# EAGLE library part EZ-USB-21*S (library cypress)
Microcontroller with USB port
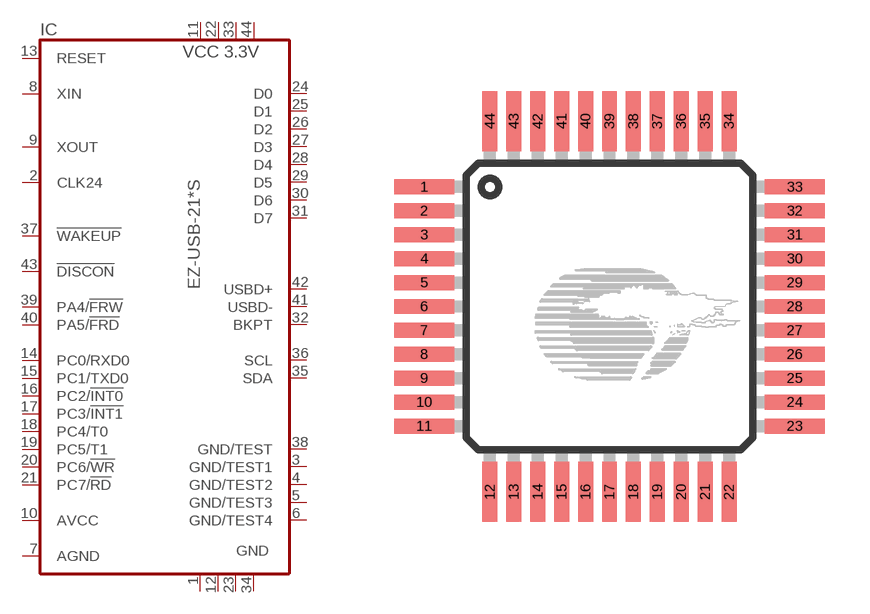
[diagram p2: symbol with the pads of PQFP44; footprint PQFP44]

Designator prefix IC

## EZ-USB-2125S (OC_FARNELL: unknown; OC_NEWARK: unknown), EZ-USB-2126S (OC_FARNELL: unknown; OC_NEWARK: unknown), EZ-USB-2135S (OC_FARNELL: unknown; OC_NEWARK: unknown), EZ-USB-2136S (OC_FARNELL: unknown; OC_NEWARK: unknown)  [PQFP44]
1  GND  pwr
2  CLK24  out
3  GND/TEST1  pwr
4  GND/TEST2  pwr
5  GND/TEST3  pwr
6  GND/TEST4  pwr
7  AGND  pwr
8  XIN  in
9  XOUT  out
10  AVCC  pwr
11  VCC3.3  pwr
12  GND  pwr
13  RESET  in
14  PC0/RXD0
15  PC1/TXD0
16  PC2/!INT0
17  PC3/!INT1
18  PC4/T0
19  PC5/T1
20  PC6/!WR
21  PC7/!RD
22  VCC3.3  pwr
23  GND  pwr
24  D0  hiz
25  D1  hiz
26  D2  hiz
27  D3  hiz
28  D4  hiz
29  D5  hiz
30  D6  hiz
31  D7  hiz
32  BKPT  out
33  VCC3.3  pwr
34  GND  pwr
35  SDA  oc
36  SCL  oc
37  !WAKEUP  in
38  GND/TEST  pwr
39  PA4/!FRW
40  PA5/!FRD
41  USBD-  hiz
42  USBD+  hiz
43  !DISCON  out
44  VCC3.3  pwr

## Footprint PQFP44 (pad centres in mm)
Plastic Quad Flat Package
smd 2 x 0.5: 1 -6.2,4; 2 -6.2,3.2; 3 -6.2,2.4; 4 -6.2,1.6; 5 -6.2,0.8; 6 -6.2,0; 7 -6.2,-0.8; 8 -6.2,-1.6; 9 -6.2,-2.4; 10 -6.2,-3.2; 11 -6.2,-4; 23 6.2,-4; 24 6.2,-3.2; 25 6.2,-2.4; 26 6.2,-1.6; 27 6.2,-0.8; 28 6.2,0; 29 6.2,0.8; 30 6.2,1.6; 31 6.2,2.4; 32 6.2,3.2; 33 6.2,4
smd 0.5 x 2: 12 -4,-6.2; 13 -3.2,-6.2; 14 -2.4,-6.2; 15 -1.6,-6.2; 16 -0.8,-6.2; 17 0,-6.2; 18 0.8,-6.2; 19 1.6,-6.2; 20 2.4,-6.2; 21 3.2,-6.2; 22 4,-6.2; 34 4,6.2; 35 3.2,6.2; 36 2.4,6.2; 37 1.6,6.2; 38 0.8,6.2; 39 0,6.2; 40 -0.8,6.2; 41 -1.6,6.2; 42 -2.4,6.2; 43 -3.2,6.2; 44 -4,6.2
